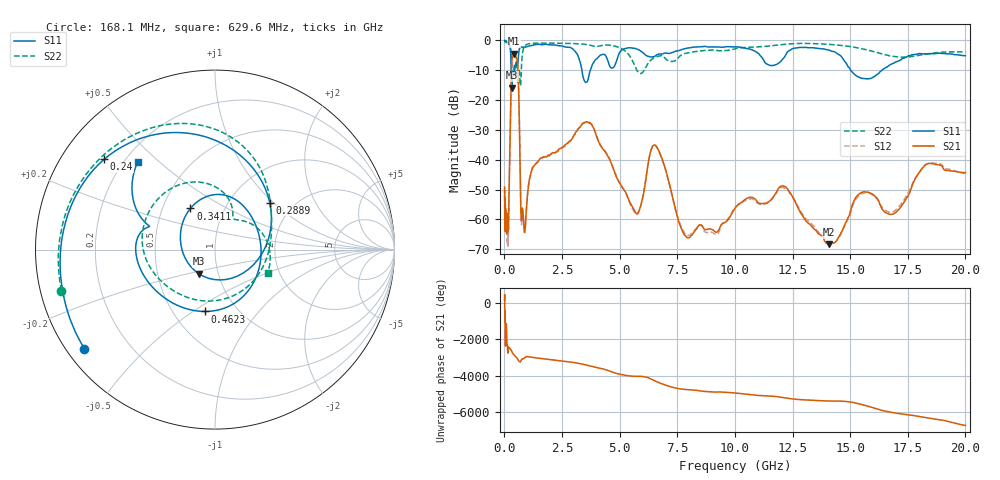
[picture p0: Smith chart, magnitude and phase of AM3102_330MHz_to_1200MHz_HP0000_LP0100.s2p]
! Date/Time: Tue, Sep 11, 2018 5:08 PM
! Network Analyzer: Agilent Technologies E8362B Rev: A.07.50.63
! Sweep from 0.010 to 20.000 GHz, 1601 Points, Sweep Type: LOG
! Power Supply: 4.950 V, 0.000 A
# Hz S DB R 50
!freq MagS11 AngS11 MagS21 AngS21 MagS12 AngS12 MagS22 AngS22
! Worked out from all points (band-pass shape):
!   1601 points, 10 MHz to 20 GHz, reference 50 ohm
!   highest |S21| = -4.41 dB at 410.6 MHz (marker M1); lowest = -68.4 dB at 14.07 GHz (marker M2)
!   |S21| within 3 dB of the highest: 319.5 MHz to 568.5 MHz (249 MHz wide, 56.1 % of centre)
!   lowest |S11| = -15.8 dB at 316.2 MHz (marker M3), VSWR 1.39, Z = 40.4 - j11.1 ohm
!   |S11| at or under -10 dB: 294.8 MHz to 444.2 MHz (149.4 MHz wide, 40.4 % of centre); 3.363 GHz to 3.729 GHz (365.6 MHz wide, 10.3 % of centre); 15.03 GHz to 16.38 GHz (1.351 GHz wide, 8.6 % of centre)
!   |S22| runs from -15.2 to -0.2 dB; largest |S21 - S12| = 0.0099
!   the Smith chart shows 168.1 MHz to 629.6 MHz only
!   S11 on the Smith chart (normalised r, x): 168.1 MHz: 0.05, -0.34; 240 MHz: 0.13, +0.35; 288.9 MHz: 1.52, +0.95; 341.1 MHz: 0.69, +0.34; 462.3 MHz: 0.71, -0.56; 629.6 MHz: 0.25, +0.43
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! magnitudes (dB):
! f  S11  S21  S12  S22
! 10 MHz  0.0  -49.2  -53.8  -0.2
! 35.55 MHz  0.0  -60.8  -61.7  -0.4
! 126.4 MHz  -0.4  -63.8  -66.1  -0.8
! 168.1 MHz  -0.8  -63.2  -65.6  -1.1
! 240 MHz  -2.0  -35.7  -35.7  -1.8
! 288.9 MHz  -7.9  -14.6  -14.7  -4.1
! 316.2 MHz  -15.8  -7.9  -7.9  -7.8
! 341.1 MHz  -11.5  -5.7  -5.8  -10.5
! 410.6 MHz  -11.8  -4.4  -4.5  -9.5
! 447.2 MHz  -9.8  -4.7  -4.7  -7.9
! 462.3 MHz  -9.1  -4.8  -4.9  -7.6
! 629.6 MHz  -3.7  -19.6  -19.6  -9.9
! 736.5 MHz  -2.2  -59.9  -61.8  -9.6
! 886.4 MHz  -2.2  -64.1  -63.7  -1.9
! 1.59 GHz  -1.4  -39.4  -39.4  -0.9
! 3.668 GHz  -11.6  -27.6  -27.3  -1.5
! 5.652 GHz  -2.6  -57.2  -57.7  -8.5
! 6.549 GHz  -5.2  -35.1  -35.4  -5.6
! 7.882 GHz  -2.7  -65.7  -65.2  -4.3
! 12.09 GHz  -6.1  -48.8  -49.3  -1.4
! 14.07 GHz  -3.2  -68.4  -67.8  -1.3
! 20 GHz  -5.1  -44.3  -44.6  -3.8
